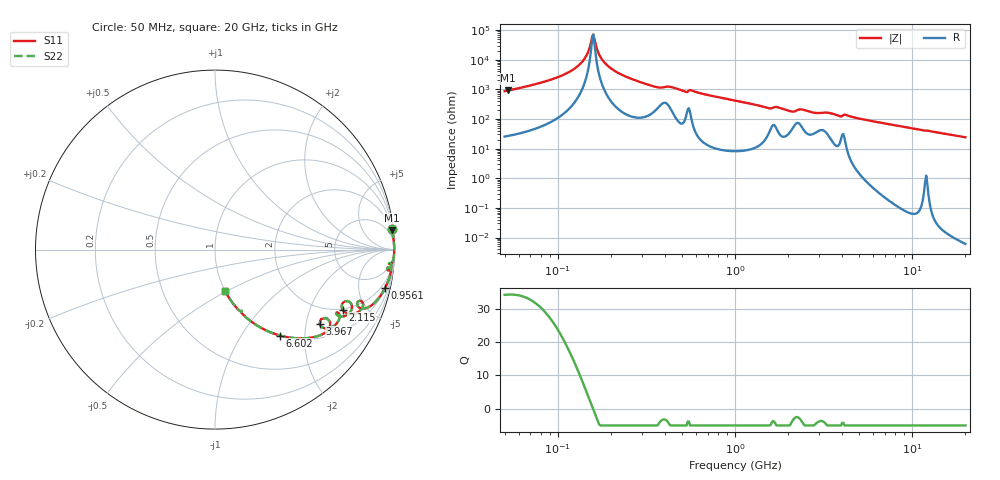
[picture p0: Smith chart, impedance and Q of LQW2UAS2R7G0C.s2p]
!Murata Part Number: LQW2UAS2R7G0C
!These Parameters are Measured in Series Mode Connection
!  o--[Z]--o
!Port1  Port2
!  o-------o
!Freq. Start=50[MHz] Stop=20[GHz], 401[Steps]
# Hz S RI R 50
!Freq.(Hz) S11(Real) S11(Imag) S21(Real) S21(Imag) S12(Real) S12(Imag) S22(Real) S22(Imag)
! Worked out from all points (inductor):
!   401 points, 50 MHz to 20 GHz, reference 50 ohm
!   read as one part in series: L = 2.47 uH near 51.52 MHz
!   highest Q = 34.2 at 52.3 MHz (marker M1), where L = 2.79 uH
!   self-resonance near 156.1 MHz
!   S11 on the Smith chart (normalised r, x): 50 MHz: 2, +17; 956.1 MHz: 1.16, -8.82; 2.115 GHz: 1.97, -3.42; 3.967 GHz: 1.41, -2.40; 6.602 GHz: 1.01, -1.51; 20 GHz: 1.00, -0.48
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5e7  0.9836 0.1131  0.0164 -0.1131  0.0164 -0.1131  0.9836 0.1131
5.229804e7  0.9852 0.1072  0.0148 -0.1072  0.0148 -0.1072  0.9852 0.1072
9.958798e7  0.9968 0.0389  0.00315 -0.0389  0.00315 -0.0389  0.9968 0.0389
1.209968e8  0.9981 0.022  0.00195 -0.022  0.00195 -0.022  0.9981 0.022
1.364002e8  0.9985 0.0121  0.00154 -0.0121  0.00154 -0.0121  0.9985 0.0121
1.448224e8  0.9986 0.00712  0.00143 -0.00712  0.00143 -0.00712  0.9986 0.00712
1.537646e8  0.9986 0.00219  0.00138 -0.00219  0.00138 -0.00219  0.9986 0.00219
1.584406e8  0.9986 -0.000273  0.00138 0.000273  0.00138 0.000273  0.9986 -0.000273
1.759554e8  0.9985 -0.00896  0.00149 0.00896  0.00149 0.00896  0.9985 -0.00896
2.013488e8  0.998 -0.0204  0.00196 0.0204  0.00196 0.0204  0.998 -0.0204
2.597386e8  0.9957 -0.0439  0.0043 0.0439  0.0043 0.0439  0.9957 -0.0439
3.721004e8  0.9742 -0.0809  0.0258 0.0809  0.0258 0.0809  0.9742 -0.0809
4.322267e8  0.9788 -0.0782  0.0212 0.0782  0.0212 0.0782  0.9788 -0.0782
9.560587e8  0.9476 -0.2138  0.0524 0.2138  0.0524 0.2138  0.9476 -0.2138
1e9  0.9421 -0.224  0.0579 0.224  0.0579 0.224  0.9421 -0.224
2.114743e9  0.7104 -0.3338  0.2896 0.3338  0.2896 0.3338  0.7104 -0.3338
2.348516e9  0.7591 -0.3024  0.2409 0.3024  0.2409 0.3024  0.7591 -0.3024
2.728004e9  0.7061 -0.373  0.2939 0.373  0.2939 0.373  0.7061 -0.373
3.967106e9  0.5829 -0.4147  0.4171 0.4147  0.4171 0.4147  0.5829 -0.4147
6.601595e9  0.3633 -0.479  0.6367 0.479  0.6367 0.479  0.3633 -0.479
7.442007e9  0.3061 -0.4596  0.6939 0.4596  0.6939 0.4596  0.3061 -0.4596
2e10  0.0554 -0.2286  0.9446 0.2286  0.9446 0.2286  0.0554 -0.2286
